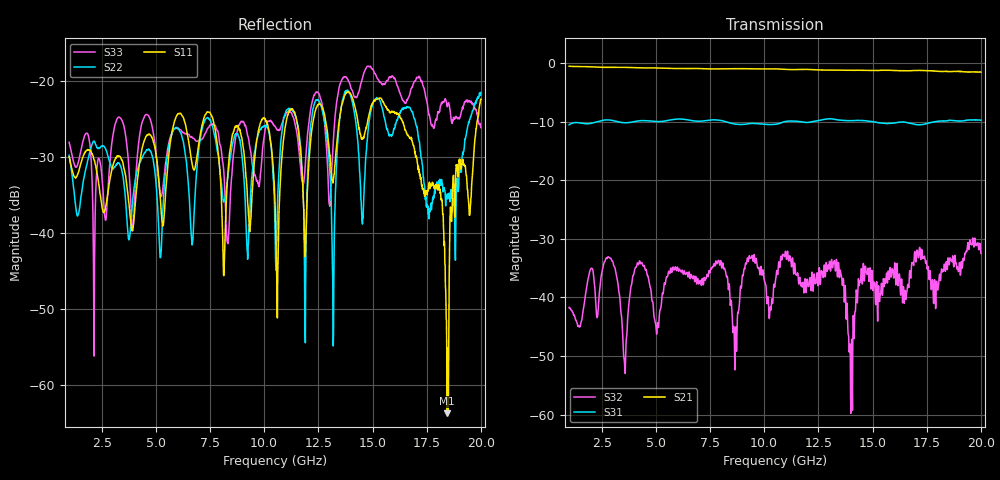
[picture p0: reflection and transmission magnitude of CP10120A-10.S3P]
! Amtery
! Email info@amtery.com
! Phone 886-2-2883-7839
! Model Number CP10120A-10
! 3-port S-parameter measurement data for Directional Coupler
! Frequency Range 1 GHz to 20 GHz
! Port 1 Input
! Port 2 Output
! Port 3 Coupled
# Hz S dB R 50
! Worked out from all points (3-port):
!   1521 points, 1 GHz to 20 GHz, reference 50 ohm
!   strongest paths, dB at 1 GHz, 5.75 GHz, 10.5 GHz, 15.25 GHz, 20 GHz:
!     S21: -0.5, -0.9, -1.0, -1.3, -1.6
!     S31: -10.6, -9.7, -10.5, -10.2, -9.8
!     S32: -41.7, -35.6, -37.8, -41.2, -32.5
!   lowest |S11| = -63.8 dB at 18.45 GHz (marker M1), VSWR 1.00, Z = 50 - j0.0458 ohm
!   |S11| at or under -10 dB: start of sweep to end of sweep
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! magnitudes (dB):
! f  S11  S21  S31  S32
! 1 GHz  -29.9  -0.5  -10.6  -41.7
! 5.213 GHz  -35.6  -0.9  -10.0  -42.0
! 7.675 GHz  -25.5  -1.0  -9.7  -34.3
! 8.312 GHz  -32.5  -1.0  -10.1  -36.7
! 10.5 GHz  -36.2  -1.0  -10.5  -37.8
! 15.38 GHz  -22.2  -1.3  -10.2  -39.3
! 18.12 GHz  -34.8  -1.5  -9.9  -37.0
! 18.45 GHz  -63.8  -1.5  -9.9  -35.3
! 18.68 GHz  -37.2  -1.5  -9.8  -33.9
! 20 GHz  -22.4  -1.6  -9.8  -32.5
